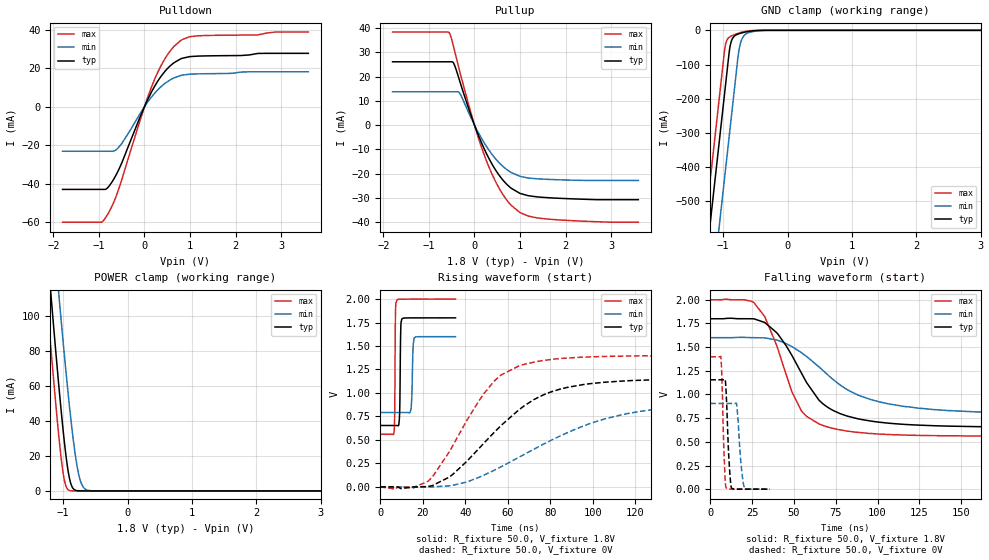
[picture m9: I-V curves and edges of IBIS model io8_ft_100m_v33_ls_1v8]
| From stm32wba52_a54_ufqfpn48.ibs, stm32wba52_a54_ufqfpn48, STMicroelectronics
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[Model]   io8_ft_100m_v33_ls_1v8
Model_type I/O
Polarity   Non-Inverting
Enable   Active-Low
| CAP_THRESHOLD on pad IOFT is "UDTCAPC" :
| Rising=30.0% of vddiom   Falling=70.0% of vddiom
| C_comp min and max val. don't necessarily correlate with the min and max pvt
| but are the smallest and greatest pad capacitance found.
| var   typ   min   max
C_comp   2.30356pF  2.19153pF  2.50006pF
|C_comp_pullup   1.45355pF  1.38790pF  1.55605pF
|C_comp_pulldown   850.01020fF  803.62502fF  944.00706fF
Vinl = 800.0mV
Vinh = 1.0V
Vmeas = 900.0mV   | Reference voltage for timing measurements
Cref  = 50.0pF   | Timing specification test load capacitance value
Rref  = 1.0MOhm   | Timing specification test load resistance value
Vref  = 990.0mV   | Timing specification test load voltage
[Model Spec]
| TIME_THRESHOLD on pin ZIV33M is "CMOS" :
| Rising=50.0% of vddiom   Falling=50.0% of vddiom
Vinl 697.50000mV 636.50000mV 765.50000mV
Vinh 1.08850V 942.50000mV 1.21750V
| variable   typ   min   max
[Temperature Range] 25.0 140.0 -40.0
| variable   typ   min   max
[Voltage Range] 1.8V 1.6V 2.0V
| variable   typ   min   max
[POWER Clamp Reference] 1.8V 1.6V 2.0V
| variable   typ   min   max
[GND Clamp Reference] 0V 0V 0V
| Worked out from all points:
|   slope of the pulldown table from 0 to 0.27 V, typ, clamps not added: 21.7 ohm
|   slope of the pullup table from 0 to 0.27 V, typ, clamps not added: 22.5 ohm
|   GND clamp passes 1 mA (typ) near -0.51 V on its own axis
|   POWER clamp passes 1 mA (typ) near -0.83 V on its own axis
|   rising waveform, R_fixture 50.0, V_fixture 1.8V: 20-80 % time 333ps typ, 525ps min, 256ps max; typ from 0.654 V to 1.8 V
|   falling waveform, R_fixture 50.0, V_fixture 1.8V: 20-80 % time 25.6ns typ, 40ns min, 18.7ns max; typ from 1.8 V to 0.654 V
|   rising waveform, R_fixture 50.0, V_fixture 0V: 20-80 % time 33.1ns typ, 51.7ns min, 23.6ns max; typ from 0 V to 1.16 V
|   falling waveform, R_fixture 50.0, V_fixture 0V: 20-80 % time 1.72ns typ, 2.26ns min, 1.41ns max; typ from 1.16 V to 0 V
[POWER Clamp]
-1.8V     396.4mA    438.1mA    365.5mA
-1.26V    143.5mA    194.6mA    112.6mA
-1.19V    112.3mA    164.2mA    81.56mA
-1.06V    57.23mA    109.3mA    28.68mA
-1.02V    41.75mA    93.06mA    15.5mA
-980mV    27.6mA     77.28mA    5.935mA
-910mV    8.693mA    51.24mA    382.3uA
-850mV    1.642mA    31.41mA    23.97uA
-760mV    69.41uA    9.714mA    358.6nA
-700mV    7.83uA     2.919mA    21.79nA
-620mV    424.6nA    410.3uA    573.9pA
3.6V      0A         0A         0A
[GND Clamp]
-1.8V     -1.583A    -1.83A     -1.456A
-1.43V    -953.9mA   -1.201A    -826.8mA
-1.24V    -630.9mA   -877.8mA   -503.8mA
-1.05V    -307.9mA   -554.8mA   -180.8mA
-970mV    -171.9mA   -418.8mA   -48.31mA
-910mV    -69.87mA   -316.8mA   -20.91mA
-880mV    -36.5mA    -265.8mA   -17.19mA
-830mV    -17.68mA   -180.8mA   -12.97mA
-750mV    -9.66mA    -53.66mA   -7.697mA
-690mV    -6.479mA   -19.19mA   -4.622mA
-600mV    -3.058mA   -6.478mA   -1.59mA
3.6V      1.279nA    1.39uA     517.2pA
| variable   typ   min   max
[Pullup Reference] 1.8V 1.6V 2.0V
| variable   typ   min   max
[Pulldown Reference] 0V 0V 0V
[Pullup]
-1.8V     26.12mA    13.77mA    38.36mA
-560mV    26.12mA    13.77mA    38.22mA
-460mV    25.58mA    13.77mA    32.35mA
-330mV    18.52mA    13.29mA    22.64mA
20mV      -1.006mA   -751.6uA   -1.259mA
280mV     -12.36mA   -9.262mA   -15.51mA
450mV     -18.1mA    -13.58mA   -22.78mA
630mV     -22.78mA   -17.1mA    -28.78mA
810mV     -26.07mA   -19.57mA   -33.13mA
1V        -28.15mA   -21.12mA   -36.04mA
1.6V      -29.9mA    -22.35mA   -38.71mA
3.6V      -30.74mA   -22.8mA    -40.02mA
[Pulldown]
-1.8V     -42.97mA   -23.15mA   -59.99mA
-950mV    -42.97mA   -23.15mA   -59.99mA
-850mV    -42.87mA   -23.15mA   -57.45mA
-670mV    -37.41mA   -23.03mA   -49.3mA
-550mV    -31.91mA   -20.61mA   -41.6mA
10mV      539.8uA    356.7uA    722uA
230mV     10.88mA    7.174mA    14.64mA
500mV     19.69mA    12.93mA    26.79mA
790mV     24.78mA    16.15mA    34.26mA
1V        26.02mA    16.89mA    36.38mA
1.18V     26.27mA    17.05mA    36.82mA
3.6V      27.7mA     18.13mA    38.74mA
[Ramp]
dV/dt_r 693.10421mV/32.97565ns 543.30231mV/51.65443ns 838.83496mV/23.2558ns
dV/dt_f 687.71572mV/25.4415ns 485.01501mV/39.82117ns 864.01188mV/18.13523ns
R_load = 50.0
| Removed startup time: 0s 0s 0s  .
| Removed end time: 35.4ns.
[Rising Waveform]
R_fixture   = 50.0
V_fixture   = 1.8V
V_fixture_min = 1.6V
V_fixture_max = 2.0V
0s        653.8mV    791.8mV    560mV
6.5ns     653.8mV    791.8mV    586.1mV
7.15ns    653.9mV    791.8mV    1.846V
7.95ns    653.7mV    791.8mV    1.994V
9.05ns    752.2mV    791.8mV    1.998V
9.6ns     1.648V     791.8mV    1.998V
10.15ns   1.788V     791.8mV    1.999V
14.45ns   1.799V     824.7mV    1.999V
15.9ns    1.799V     1.585V     1.999V
35.4ns    1.8V       1.6V       2V
| Removed startup time: 0s 0s 0s  .
| Removed end time: 398.4ns.
[Falling Waveform]
R_fixture   = 50.0
V_fixture   = 1.8V
V_fixture_min = 1.6V
V_fixture_max = 2.0V
0s        1.8V       1.6V       2V
26.15ns   1.799V     1.6V       1.969V
32.55ns   1.76V      1.598V     1.822V
39.55ns   1.655V     1.576V     1.525V
54.4ns    1.229V     1.443V     828.8mV
64.9ns    941.9mV    1.293V     690.3mV
77.6ns    798mV      1.1V       625.2mV
102.8ns   704.1mV    914.4mV    580.9mV
142.8ns   665.8mV    829.3mV    563.5mV
398.4ns   653.8mV    791.6mV    560mV
| Removed startup time: 0s 0s 0s  .
| Removed end time: 398.35ns.
[Rising Waveform]
R_fixture   = 50.0
V_fixture   = 0V
V_fixture_min = 0V
V_fixture_max = 0V
0s        4.767nV    680.3nV    4.106nV
22.3ns    3.291mV    -59.15uV   57.66mV
34.35ns   138.2mV    18.53mV    449.4mV
46.65ns   414.3mV    104mV      924.1mV
53.95ns   588.7mV    181.2mV    1.134V
65.05ns   817.5mV    313.3mV    1.286V
76.7ns    978.8mV    454mV      1.347V
105.7ns   1.115V     724.9mV    1.389V
149ns     1.15V      863.5mV    1.398V
398.4ns   1.155V     905.5mV    1.398V
| Removed startup time: 0s 0s 0s  .
| Removed end time: 35.4ns.
[Falling Waveform]
R_fixture   = 50.0
V_fixture   = 0V
V_fixture_min = 0V
V_fixture_max = 0V
0s        1.155V     905.4mV    1.398V
6.3ns     1.155V     905.4mV    1.399V
8ns       1.155V     905.4mV    479.5mV
9.4ns     1.052V     905.4mV    17.27mV
10.85ns   414.1mV    905.4mV    2.116mV
12.55ns   20.03mV    905.4mV    864.4uV
15.9ns    799.6uV    878.8mV    484.6uV
18.1ns    439.9uV    321.3mV    411.9uV
20.4ns    345.2uV    18.4mV     379.1uV
35.4ns    324.2uV    245.4uV    260.7uV
